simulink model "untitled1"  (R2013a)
settings: Solver=ode23t  StartTime=0.0  StopTime=100  RelTol=1e-3
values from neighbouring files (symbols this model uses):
  m = v*BEAM.rho    [FlexBeamModelConstruct2.m]    (also in FlexBeamModelConstruct3.m = BEAM.rho*v; FlexBeam_1D_Construct.m = REF.m/REF.l*a.*(linspace(1-OPT.MassBiais+1e-6,1+OPT.MassBiai; FlexBeam_3D_Construct.m = REF.m/REF.l*a.*(linspace(1-OPT.MassBiais+1e-6,1+OPT.MassBiai)
  N = D(1)+(H4^2+H3^2)/H2^2-(E(1)*H4+F(1)*H3)/H2    [MGD.m]    (also in MGD2.m)
  s = [-sign(imag(KGZ_fr_tmp(1:wLimID_tmp-1))-imag(Margin.c(1)));                         -sign(imag(KGZ_fr_tmp(wLimID_tmp:end))-imag(Margin.c(2)))]    [RO_EX1_sub_21.m]    (also in LinprogReguliOptimFunc_1.m = -sign(imag(KGZ_fr_tmp)); LinprogReguliOptimFunc_2.m = -sign(imag(KGZ_fr_tmp)); LinprogReguliOptimFunc_1 - Copie.m = -sign(imag(KGZ_fr_tmp)))
undefined symbols (not defined in the file or in its folder): deg, kg
libraries: mblibv1 x12, simulink x1

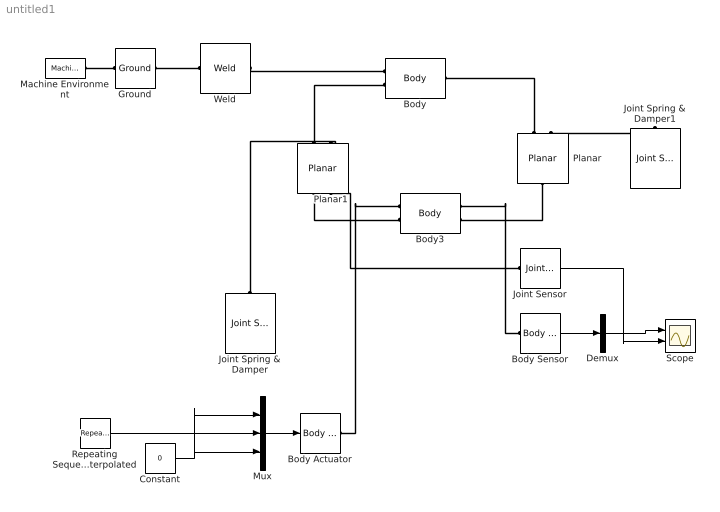
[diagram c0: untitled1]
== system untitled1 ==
  Body : mblibv1/Bodies/Body  LConnTagsString=CS3|CS1  RConnTagsString=CS2  UpdateFromCAD=off  DialogClass=MechanicalBodyBlock  Mass=3  MassUnits=kg  InertiaUnits=kg*m^2  Inertia=2/3*eye(3)  Shape=Cylinder  ShapeDims=[1 1]  ShapeUnits=m  ShapeUse=false  Density=1  DensityUnits=kg/m^3  DensityUse=false  GraphicsMode=MACHINE_DEFAULT  BodyColorSelMode=MACHINE_DEFAULT  BodyColor=[1 0 0]  AttachedToCS=CG  CG=Left$CG$[0 0 0]$World$World$m$[0 0 0]$Euler X-Y-Z$deg$WORLD$false$none  WorkingFrames=Left$CS3$[0 0 0]$CG$CG$m$[0 0 0]$Euler X-Y-Z$deg$WORLD$true$none#Left$CS1$[-5/3 0 0]$CG$CG$m$[0 0 0]$Euler X-Y-Z$deg$WORLD$true$none#Right$CS2$[4/3 0 0]$CG$CG$m$[0 0 0]$Euler X-Y-Z$deg$WORLD$true$none  CGPos=[0 0 0]  CGRot=[0 0 0]  CS0Pos=[]  CS0Rot=[]  CS1Pos=[-5/3 0 0]  CS1Rot=[0 0 0]  CS2Pos=[4/3 0 0]  CS2Rot=[0 0 0]  CS3Pos=[0 0 0]  CS3Rot=[0 0 0]  CS4Pos=[]  CS4Rot=[]  CS5Pos=[]  CS5Rot=[]  CS6Pos=[]  CS6Rot=[]  CS7Pos=[]  CS7Rot=[]  CS8Pos=[]  CS8Rot=[]  CS9Pos=[]  CS9Rot=[]  CS10Pos=[]  CS10Rot=[]  CS11Pos=[]  CS11Rot=[]  CS12Pos=[]  CS12Rot=[]  CS13Pos=[]  CS13Rot=[]  CS14Pos=[]  CS14Rot=[]  CS15Pos=[]  CS15Rot=[]  CS16Pos=[]  CS16Rot=[]  CS17Pos=[]  CS17Rot=[]  CS18Pos=[]  CS18Rot=[]  CS19Pos=[]  CS19Rot=[]  CS20Pos=[]  CS20Rot=[]
  Body Actuator : mblibv1/Sensors &  Actuators/Body Actuator  UpdateFromCAD=off  PhysicalDomain=Mechanical  PortType=blob  ActuationStyle=Force  AngleUnits=deg  ArcVelocityUnits=deg/s  ArcAccelerationUnits=deg/s^2  CoordPositionUnits=m  VelocityUnits=m/s  AccelerationUnits=m/s^2  ForceUnits=N  TorqueUnits=N*m  ActiveIO=on  Width=3  DialogClass=MechanicalActuatorBlock  ReferenceFrame=Absolute (World)  Angle=off  CoordPosition=on  Force=on  Torque=off
  Body Sensor : mblibv1/Sensors &  Actuators/Body Sensor  UpdateFromCAD=off  PhysicalDomain=Mechanical  PortType=blob  Muxed=on  Pose=off  Angle=on  AngleUnits=deg  ArcVelocity=off  ArcVelocityUnits=deg/s  ArcAcceleration=off  ArcAccelerationUnits=deg/s^2  CoordPosition=on  CoordPositionUnits=m  Velocity=off  VelocityUnits=m/s  Acceleration=off  AccelerationUnits=m/s^2  Quaternion=on  QuaternionDT=off  QuaternionDDT=off  QuaternionUnits=off  OutputVector=[1]  ActiveIO=on  Width=3  DialogClass=MechanicalSensorBlock  ReferenceFrame=Absolute (World)
  Body3 : mblibv1/Bodies/Body  LConnTagsString=CS3|CS1  RConnTagsString=CS4|CS2  UpdateFromCAD=off  DialogClass=MechanicalBodyBlock  Mass=3  MassUnits=kg  InertiaUnits=kg*m^2  Inertia=2/3*eye(3)  Shape=Cylinder  ShapeDims=[1 1]  ShapeUnits=m  ShapeUse=false  Density=1  DensityUnits=kg/m^3  DensityUse=false  GraphicsMode=MACHINE_DEFAULT  BodyColorSelMode=MACHINE_DEFAULT  BodyColor=[1 0 0]  AttachedToCS=CG  CG=Left$CG$[0 0 0]$World$World$m$[0 0 0]$Euler X-Y-Z$deg$WORLD$false$none  WorkingFrames=Right$CS4$[0 0 0]$CG$CG$m$[0 0 0]$Euler X-Y-Z$deg$WORLD$true$none#Left$CS3$[0 0 0]$CG$CG$m$[0 0 0]$Euler X-Y-Z$deg$WORLD$true$none#Left$CS1$[-5/3 0 0]$CG$CG$m$[0 0 0]$Euler X-Y-Z$deg$WORLD$true$none#Right$CS2$[4/3 0 0]$CG$CG$m$[0 0 0]$Euler X-Y-Z$deg$WORLD$true$none  CGPos=[0 0 0]  CGRot=[0 0 0]  CS0Pos=[]  CS0Rot=[]  CS1Pos=[-5/3 0 0]  CS1Rot=[0 0 0]  CS2Pos=[4/3 0 0]  CS2Rot=[0 0 0]  CS3Pos=[0 0 0]  CS3Rot=[0 0 0]  CS4Pos=[0 0 0]  CS4Rot=[0 0 0]  CS5Pos=[]  CS5Rot=[]  CS6Pos=[]  CS6Rot=[]  CS7Pos=[]  CS7Rot=[]  CS8Pos=[]  CS8Rot=[]  CS9Pos=[]  CS9Rot=[]  CS10Pos=[]  CS10Rot=[]  CS11Pos=[]  CS11Rot=[]  CS12Pos=[]  CS12Rot=[]  CS13Pos=[]  CS13Rot=[]  CS14Pos=[]  CS14Rot=[]  CS15Pos=[]  CS15Rot=[]  CS16Pos=[]  CS16Rot=[]  CS17Pos=[]  CS17Rot=[]  CS18Pos=[]  CS18Rot=[]  CS19Pos=[]  CS19Rot=[]  CS20Pos=[]  CS20Rot=[]
  Constant : Constant  Value=0
  Demux : Demux  Outputs=3
  Ground : mblibv1/Bodies/Ground  UpdateFromCAD=off  LeftPortType=env  RightPortType=workingframe  PhysicalDomain=Mechanical  DialogClass=GroundBlock  CoordPosition=[0 0 0]  CoordPositionUnits=m  StateVectorMgrId=0  MachineId=[1 0]  ShowEnvPort=on
  Joint Sensor : mblibv1/Sensors &  Actuators/Joint Sensor  UpdateFromCAD=off  PhysicalDomain=Mechanical  PortType=blob  Muxed=on  Pose=off  Angle=on  AngleUnits=rad  ArcVelocity=off  ArcVelocityUnits=deg/s  ArcAcceleration=off  ArcAccelerationUnits=deg/s^2  CoordPosition=off  CoordPositionUnits=m  Velocity=off  VelocityUnits=m/s  Acceleration=off  AccelerationUnits=m/s^2  Quaternion=on  QuaternionDT=off  QuaternionDDT=off  QuaternionUnits=off  OutputVector=[1]  ActiveIO=on  Width=1  DialogClass=MechanicalSensorBlock  Primitive=R1  Force=off  ForceUnits=N  Torque=off  TorqueUnits=N*m  ReferenceFrame=Absolute (World)  ReactionSensedSide=Base  ReactionReferenceFrame=Absolute (World)  ReactionForce=off  ReactionForceUnits=N  ReactionMoment=off  ReactionMomentUnits=N*m
  Joint Spring & Damper : mblibv1/Force  Elements/Joint Spring & Damper  UpdateFromCAD=off  DialogClass=JointSpringDamper  JFEParameters=P1$true$10$0.0001$0$m$m/s$N$deg$deg/s$N*m#P2$true$1$0.0001$0$m$m/s$N$deg$deg/s$N*m#P3$false$0$0$0$m$m/s$N$deg$deg/s$N*m#R1$true$0.0001$0.0001$0$m$m/s$N$deg$deg/s$N*m#R2$false$0$0$0$m$m/s$N$deg$deg/s$N*m#R3$false$0$0$0$m$m/s$N$deg$deg/s$N*m#S$false$0$0$0$m$m/s$N$deg$deg/s$N*m
  Joint Spring & Damper1 : mblibv1/Force  Elements/Joint Spring & Damper  UpdateFromCAD=off  DialogClass=JointSpringDamper  JFEParameters=P1$true$10$0.0001$0$m$m/s$N$deg$deg/s$N*m#P2$true$1$0.0001$0$m$m/s$N$deg$deg/s$N*m#P3$false$0$0$0$m$m/s$N$deg$deg/s$N*m#R1$true$0.0001$0.0001$0$m$m/s$N$deg$deg/s$N*m#R2$false$0$0$0$m$m/s$N$deg$deg/s$N*m#R3$false$0$0$0$m$m/s$N$deg$deg/s$N*m#S$false$0$0$0$m$m/s$N$deg$deg/s$N*m
  Machine Environment : mblibv1/Bodies/Machine Environment  PortType=env  PhysicalDomain=Mechanical  DialogTemplateClass=MECH.MachineEnvironment  SyncWhenCopied=off  Gravity=[0 0 0]  GravityUnits=m/s^2  GravityAsSignal=off  Dimensionality=Auto-detect  AnalysisType=Forward dynamics  LinearAssemblyTolerance=1e-3  LinearAssemblyToleranceUnits=m  AngularAssemblyTolerance=1e-3  AngularAssemblyToleranceUnits=rad  ConstraintSolverType=Stabilizing  ConstraintRelTolerance=1e-4  ConstraintAbsTolerance=1e-4  UseRobustSingularityHandling=off  RedundancyAnalysisToleranceType=Automatically select tolerance  RedundancyAnalysisTolerance=1e-14  StatePerturbationType=Fixed  PerturbationSize=1e-5  VisualizeMachine=on  BodyVisualizationType=Use model default body geometries  BodyColorSelMode=Use model default  DefaultBodyColor=[1 0 0]
  Mux : Mux  Inputs=3
  Planar : mblibv1/Joints/Planar  LConnTagsString=__newl0|SA1  RConnTagsString=__newr0  UpdateFromCAD=off  NumSAPorts=1  CutJoint=off  MarkAsCut=off  Primitives=prismatic_prismatic  PrimitiveProps=P1$World$[1 0 0]$prismatic#P2$World$[0 1 0]$prismatic#R1$World$[0 0 1]$revolute  DialogClass=JointBlock  P1Axis=[1 0 0]  P2Axis=[0 1 0]  R1Axis=[0 0 1]
  Planar1 : mblibv1/Joints/Planar  LConnTagsString=__newl0|SA1  RConnTagsString=__newr0|SA1  UpdateFromCAD=off  NumSAPorts=2  CutJoint=off  MarkAsCut=off  Primitives=prismatic_prismatic  PrimitiveProps=P1$World$[1 0 0]$prismatic#P2$World$[0 1 0]$prismatic#R1$World$[0 0 1]$revolute  DialogClass=JointBlock  P1Axis=[1 0 0]  P2Axis=[0 1 0]  R1Axis=[0 0 1]
  Repeating Sequence Interpolated : simulink/Sources/Repeating Sequence Interpolated  OutValues=[0 0 1 1 0 0].'  TimeValues=[0 1 1.1 1.2 1.3 100 ].'  LookUpMeth=Interpolation-Use End Values  tsamp=0.01  OutMin=[]  OutMax=[]  OutDataTypeStr=double  OutputDataTypeScalingMode=double  OutDataType=fixdt(0,8)  OutScaling=2^-10
  Scope : Scope  NumInputPorts=2
  Weld : mblibv1/Joints/Weld  LConnTagsString=__newl0  RConnTagsString=__newr0  UpdateFromCAD=off  NumSAPorts=0  CutJoint=off  MarkAsCut=off  Primitives=weld  PrimitiveProps=W$WORLD$[0 0 0]$weld  DialogClass=JointBlock  WAxis=[0 0 0]
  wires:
  Mux/1 -> Body Actuator/1
  Constant/1 -> Mux/3, Mux/1
  Body Sensor/1 -> Demux/1
  Demux/2 -> Scope/1
  Joint Sensor/1 -> Scope/2
  Repeating Sequence Interpolated/1 -> Mux/2
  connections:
  Machine Environment/RConn1 -- Ground/LConn1
  Weld/LConn1 -- Ground/RConn1
  Weld/RConn1 -- Body/LConn1
  Planar/LConn1 -- Body/RConn1
  Planar/RConn1 -- Body3/RConn2
  Joint Spring & Damper/LConn1 -- Planar1/LConn2
  Joint Spring & Damper1/LConn1 -- Planar/LConn2
  Body Actuator/RConn1 -- Body3/LConn1
  Body Sensor/LConn1 -- Body3/RConn1
  Joint Sensor/LConn1 -- Planar1/RConn2
  Planar1/LConn1 -- Body/LConn2
  Planar1/RConn1 -- Body3/LConn2
